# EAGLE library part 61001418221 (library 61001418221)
WURTH ELEKTRONIK - 61001418221 - Board-To-Board Connector, 2.54 mm, 14 Contacts, Header, WR-PHD Series, Surface Mount, 1 Rows Source: Datasheet
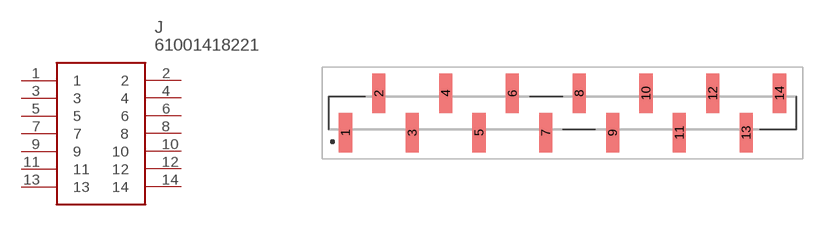
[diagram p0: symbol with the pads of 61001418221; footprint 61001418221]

Designator prefix J

## 61001418221 (Description: WURTH ELEKTRONIK - 61001418221 - Board-To-Board Connector, 2.54 mm, 14 Contacts, Header, WR-PHD Series, Surface Mount, 1 Rows; Height: 9.3mm; Manufacturer_Name: Wurth Elektronik; Manufacturer_Part_Number: 61001418221; Mouser_Part_Number: 710-61001418221; Mouser_Price-Stock: https://www.mouser.co.uk/ProductDetail/Wurth-Elektronik/61001418221?qs=PhR8RmCirEZbaE9NVx%2FAsQ%3D%3D)  [61001418221]
1  1
2  2
3  3
4  4
5  5
6  6
7  7
8  8
9  9
10  10
11  11
12  12
13  13
14  14

## Footprint 61001418221 (pad centres in mm)
61001418221-1
smd 1 x 3: 1 -16.51,-1.5; 2 -13.97,1.5; 3 -11.43,-1.5; 4 -8.89,1.5; 5 -6.35,-1.5; 6 -3.81,1.5; 7 -1.27,-1.5; 8 1.27,1.5; 9 3.81,-1.5; 10 6.35,1.5; 11 8.89,-1.5; 12 11.43,1.5; 13 13.97,-1.5; 14 16.51,1.5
